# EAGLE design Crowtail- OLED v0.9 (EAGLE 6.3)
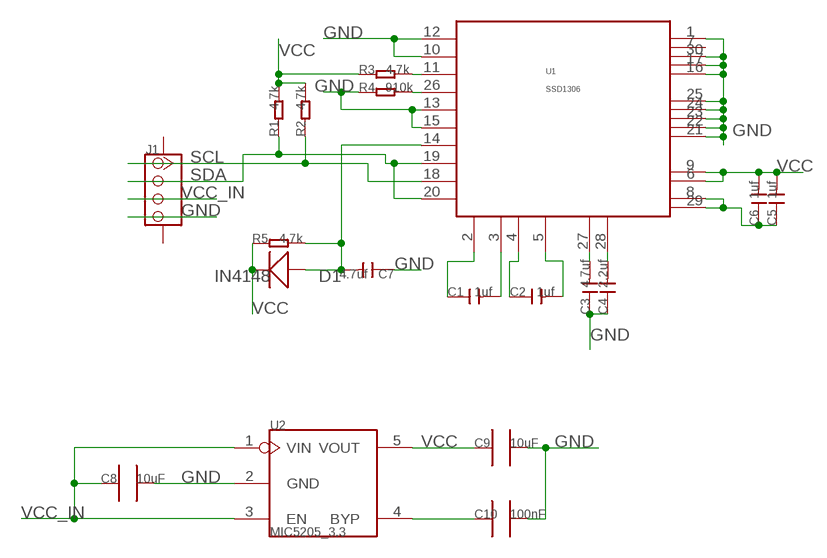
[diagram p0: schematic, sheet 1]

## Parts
C1  1uf  C-0603  [C0603]
C2  1uf  C-0603  [C0603]
C3  4.7uf  C-0603  [C0603]
C4  2.2uf  C-0603  [C0603]
C5  1uf  C-0603  [C0603]
C6  1uf  C-0603  [C0603]
C7  4.7uf  C-0603  [C0603]
C8  10uF  C0805_S  [0805_S]
C9  10uF  C0805_S  [0805_S]
C10  100nF  C0603_S  [0603_S]
D1  IN4148  D'0805'  [SOD323]
J1  TWIG-4P-2.0-SMD-FEMALE-REINFORCE'DD'  [4P-SMD-2.0]
R1  4.7k  R-0603  [R0603]
R2  4.7k  R-0603  [R0603]
R3  4.7k  R-0603  [R0603]
R4  910k  R-0603  [R0603]
R5  4.7k  R-0603  [R0603]
U1  SSD1306  [SSD1306]
U2  MIC5205_3.3  MIC5025_X.X  [SOT23-5]

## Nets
GND: C3.1 C4.1 C7.1 C8.2 C9.2 C10.2 J1.4 R4.1 U1.1(NC_1) U1.10(BS0) U1.12(BS2) U1.13(CS#) U1.15(D/C#) U1.16(R/W#) U1.17(E/RD#) U1.21(D3) U1.22(D4) U1.23(D5) U1.24(D6) U1.25(D7) U1.30(NC_3) U2.2(GND)
N$1: R3.2 U1.11(BS1)
N$2: R4.2 U1.26(IREF)
N$3: C1.2 U1.3(C2N)
N$4: C7.2 D1.+ R5.2 U1.14(RES#)
N$5: C1.1 U1.2(C2P)
N$6: C2.1 U1.4(C1P)
N$7: C2.2 U1.5(C1N)
N$8: C3.2 U1.27(VCOMH)
N$9: C4.2 U1.28(VCC)
N$10: C10.1 U2.4(BYP)
N$11: C5.1 C6.1 U1.8(VSS) U1.29(VLSS)
SCL: J1.1 R2.1 U1.18(D0)
SDA: J1.2 R1.1 U1.19(D1) U1.20(D2)
VCC: C5.2 C6.2 C9.1 D1.- R1.2 R2.2 R3.1 R5.1 U1.6(VBAT) U1.9(VDD) U2.5(VOUT)
VCC_IN: C8.1 J1.3 U2.1(VIN) U2.3(EN)
Unconnected: J1.SS1 J1.SS2 U1.7(NC_2)

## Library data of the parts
C1-C7 = Discrete:C*: Ceramic Capacitors
C8 C9 = CPT_SMD:C0805
C10 = CPT_SMD:C0603
D1 = Discrete:D*
J1 = Connector:TWIG-4P-2.0-SMD-FEMALE-REINFORCE
R1-R5 = Discrete:R*
U1 = IC:SSD1306
U2 = ICs_v54:MIC5025_X.X

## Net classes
0 default: width 0.203 mm, drill 0.305 mm, clearance 0.203 mm

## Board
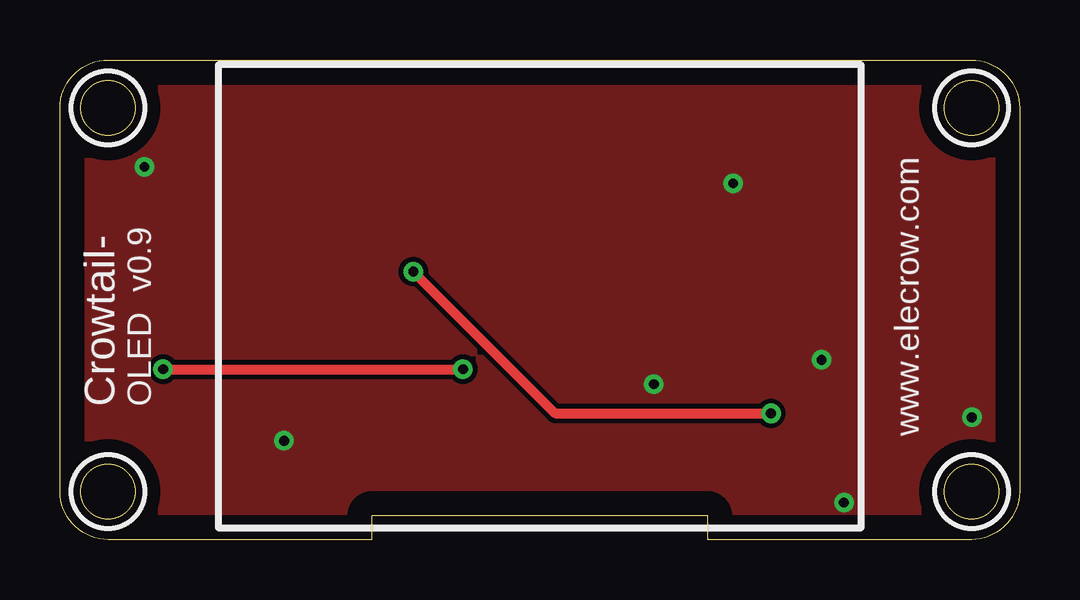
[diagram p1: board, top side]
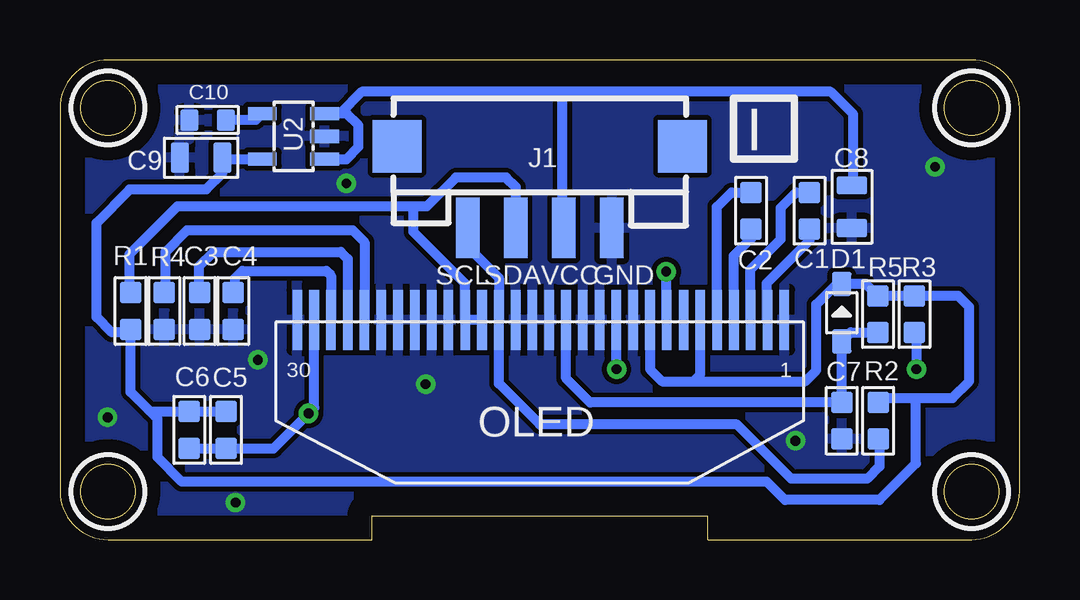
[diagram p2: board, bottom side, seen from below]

Size 40 x 20 mm. Coordinates in mm from the lower left corner, seen from the top.
Outline: 13,0 2,0 arc-90 0,2 0,18 arc-90 2,20 38,20 arc-90 40,18 40,2 arc-90 38,0 27,0 27,1 13,1 13,0
Outline: circle at 38,18 radius 1.14
Outline: circle at 2,18 radius 1.14
Outline: circle at 38,2 radius 1.14
Outline: circle at 2,2 radius 1.14
Copper layers (1*16): Top 0.035mm / dielectric 1.5mm / Bottom 0.035mm
Design rules "default *": minimum track width 10mil, minimum drill 24mil, track to track 8mil, track to pad 8mil, pad to pad 8mil, via to via 8mil, smd to smd 8mil, copper to edge 40mil, drill to drill 8mil, minimum pad ring 10mil, minimum via ring 8mil, stop-mask expansion 4mil, vias tented up to drill 100mil, thermal gap 10mil
tRestrict: area 36.5,16.5 to 39.5,19.5; area 0.5,16.5 to 3.5,19.5; area 36.5,0.5 to 39.5,3.5; area 0.5,0.5 to 3.5,3.5
bRestrict: area 36.5,16.5 to 39.5,19.5; area 0.5,16.5 to 3.5,19.5; area 36.5,0.5 to 39.5,3.5; area 0.5,0.5 to 3.5,3.5

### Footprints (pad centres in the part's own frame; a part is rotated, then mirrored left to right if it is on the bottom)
C0603 = smd 0.889 x 0.889: 1 -0.762,0; 2 0.762,0
0805_S = smd 0.762 x 1.27: 1 -0.889,0; 2 0.889,0
0603_S = smd 0.762 x 0.889: 1 -0.762,0; 2 0.762,0
SOD323 = smd 1 x 0.8: + -1.2,0; - 1.2,0
4P-SMD-2.0 = smd 0.965 x 2.54: 1 -3,0; 2 -1,0; 3 1,0; 4 3,0 | smd 2.032 x 2.184: SS1 -5.946,3.4; SS2 5.946,3.4
R0603 = smd 0.889 x 0.889: 1 -0.762,0; 2 0.762,0
SSD1306 = smd 0.4 x 2.5: 1 -10.094,-0.115; 2 -9.394,-0.115; 3 -8.694,-0.115; 4 -7.994,-0.115; 5 -7.294,-0.115; 6 -6.594,-0.115; 7 -5.894,-0.115; 8 -5.194,-0.115; 9 -4.494,-0.115; 10 -3.794,-0.115; 11 -3.094,-0.115; 12 -2.394,-0.115; 13 -1.694,-0.115; 14 -0.994,-0.115; 15 -0.294,-0.115; 16 0.406,-0.115; 17 1.106,-0.115; 18 1.806,-0.115; 19 2.506,-0.115; 20 3.206,-0.115; 21 3.906,-0.115; 22 4.606,-0.115; 23 5.306,-0.115; 24 6.006,-0.115; 25 6.706,-0.115; 26 7.406,-0.115; 27 8.106,-0.115; 28 8.806,-0.115; 29 9.506,-0.115; 30 10.206,-0.115
SOT23-5 = smd 0.55 x 1.2: 1 -0.95,-1.3; 2 0,-1.3; 3 0.95,-1.3; 4 0.95,1.3; 5 -0.95,1.3

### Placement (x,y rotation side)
C1  8.76,13.72 90 bottom
C2  11.19,13.72 90 bottom
C3  34.18,9.53 90 bottom
C4  32.77,9.53 90 bottom
C5  33.08,4.57 90 bottom
C6  34.61,4.57 90 bottom
C7  7.41,4.95 90 bottom
C8  6.98,13.88 270 bottom
C9  34.11,15.92 180 bottom
C10  33.84,17.49 180 bottom
D1  7.41,9.46 90 bottom
J1  20,13 0 bottom
R1  37.05,9.53 270 bottom
R2  5.89,4.95 90 bottom
R3  4.38,9.4 270 bottom
R4  35.65,9.53 90 bottom
R5  5.9,9.4 270 bottom
U1  19.9,9.05 180 bottom
U2  30.27,16.81 90 bottom

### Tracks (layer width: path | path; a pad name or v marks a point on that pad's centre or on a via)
GND  (via drill 0.41)
  other vias: 9.34,4.11 24.76,6.48 31.75,7.49 3.53,15.54 28.06,14.86 38.01,5.1 32.68,1.54
  pour Bottom: 40.51,21.45 -1.45,21.45 -1.45,-0.38 40.63,-0.38
  pour Top: 40.52,21.34 -1.1,21.34 -1.1,-0.29 40.52,-0.29
N$1  (via drill 0.41)
  Top 0.406: v4.3,7.1 v16.8,7.1
  Bottom 0.406: R3.2 4.3,8.56 v4.3,7.1 | v16.8,7.1 v16.81,7.11 U1.11
N$2
  Bottom 0.406: R4.2 35.6,10.34 35.6,12 34.7,12.9 27.8,12.9 27.31,12.41 U1.26
N$3
  Bottom 0.406: U1.3 11.22,9.18 11.22,11.25 9.95,12.52 9.95,13.84 9.32,14.48 C1.2
N$4
  Bottom 0.406: U1.14 18.91,6.72 17.9,5.71 C7.2 D1.+ 7.04,8.64 R5.2
N$5
  Bottom 0.406: U1.2 10.54,9.2 10.54,10.69 8.76,12.47 C1.1
N$6
  Bottom 0.406: U1.4 11.91,11.84 11.19,12.55 C2.1
N$7
  Bottom 0.406: U1.5 12.62,13.87 12.01,14.48 C2.2
N$8
  Bottom 0.406: C3.2 34.2,10.31 34.2,11.4 33.6,12 28.3,12 28.01,11.71 U1.27
N$9
  Bottom 0.406: C4.2 32.7,10.37 32.7,10.9 32.4,11.2 28.9,11.2 28.71,11.01 U1.28
N$10
  Bottom 0.406: U2.4 31.84,17.49 C10.1
N$11  (via drill 0.41)
  Top 0.406: v14.73,11.18 20.64,5.26 v29.64,5.26
  Bottom 0.406: C6.1 C5.1 31.1,3.8 v29.64,5.26 29.41,5.49 U1.29 | U1.8 14.73,9.19 v14.73,11.18
SCL
  Bottom 0.406: J1.1 22.98,12.98 22.98,12.19 21.71,10.92 U1.18 21.71,6.51 20,4.8 11.78,4.8 9.52,2.54 6.34,2.54 5.84,3.05 5.84,4.14 R2.1
SDA
  Bottom 0.406: R1.1 37.1,10.29 37.1,11.9 35.1,13.9 25.27,13.9 | 25.27,13.9 24.7,13.9 23.5,15.1 21.4,15.1 21,14.7 J1.2 | U1.19 U1.20 23.11,10.67 25.27,12.83 25.27,13.9
VCC
  Bottom 0.406: C6.2 C5.2 | C6.2 34.67,5.4 | R2.2 5.7,5.9 4.31,5.9 | 4.31,5.9 2.8,5.9 2.1,6.6 2.1,9.7 2.56,10.16 R3.1 R5.1 6.41,10.66 D1.- | R1.2 37.17,8.6 | U1.9 15.4,7.1 14.9,6.6 13.6,6.6 | 13.6,6.6 13.31,6.89 U1.6 | D1.- | 4.31,5.9 4.31,3.17 5.84,1.65 9.77,1.65 10.54,2.41 34.92,2.41 35.94,3.43 35.94,5.04 36.23,5.33 | 36.23,5.33 37.05,6.15 R1.2 | 36.23,5.33 C6.2 | U2.5 33.17,15.86 C9.1 33.23,15.28 33.9,14.61 37.08,14.61 | 37.09,14.61 37.08,14.61 | R1.2 37.13,8.64 37.84,8.64 38.48,9.27 38.48,13.21 37.08,14.61 | 13.6,6.6 8.94,6.6 8.48,7.06 8.48,9.8 7.62,10.66 D1.-
VCC_IN
  Bottom 0.406: U2.3 28.95,17.78 | J1.3 19.05,13.04 19.05,18.67 | U2.3 28.33,17.76 27.43,18.67 19.05,18.67 | 19.05,18.67 7.87,18.67 6.93,17.73 6.93,14.82 C8.1 | U2.1 28.06,15.86 28.06,15.88 27.55,16.38 27.55,17.27 28.05,17.76 U2.3

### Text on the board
tPlace: v0.9 | Crowtail- | OLED | www.elecrow.com
bPlace: I | GND | VCC | SDA | SCL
